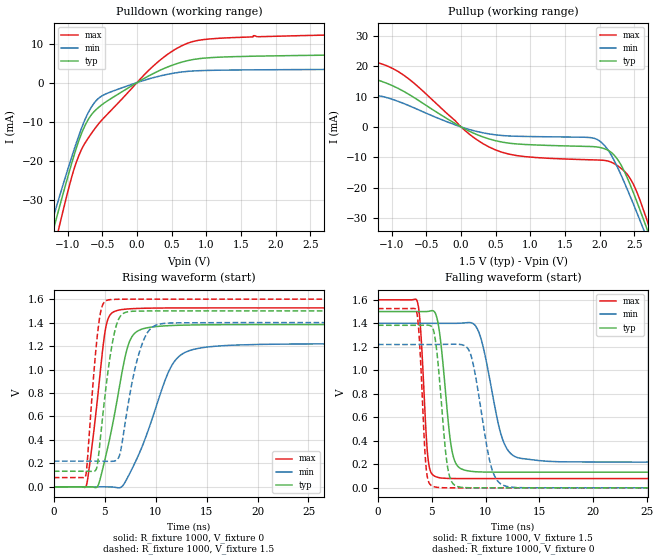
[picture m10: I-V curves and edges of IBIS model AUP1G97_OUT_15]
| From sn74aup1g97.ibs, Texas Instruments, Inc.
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[Model]   AUP1G97_OUT_15
Model_type  Output
Vref =   0
Rref =   1E6
Cref =   30p
Vmeas =   0.75
| variable   typ   min   max
C_comp   2.79pF   1.99pF   4.00pF
| C_pullup   3.03pF   1.99pF   4.00pF
| C_pulldown   2.56pF   2.15pF   3.05pF
[Temperature Range]   40   100   -40
| Ambient temperature   25   85   -40
[Voltage range]   1.5   1.4   1.6
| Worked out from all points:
|   slope of the pulldown table from 0 to 0.225 V, typ, clamps not added: 101 ohm
|   slope of the pullup table from 0 to 0.225 V, typ, clamps not added: 90.4 ohm
|   rising waveform, R_fixture 1000, V_fixture 0: 20-80 % time 1.86ns typ, 3.07ns min, 1.18ns max; typ from 0 V to 1.38 V
|   falling waveform, R_fixture 1000, V_fixture 1.5: 20-80 % time 873ps typ, 1.57ns min, 528ps max; typ from 1.5 V to 0.133 V
|   rising waveform, R_fixture 1000, V_fixture 1.5: 20-80 % time 1.19ns typ, 1.61ns min, 854ps max; typ from 0.133 V to 1.5 V
|   falling waveform, R_fixture 1000, V_fixture 0: 20-80 % time 790ps typ, 1.33ns min, 489ps max; typ from 1.38 V to 0 V
[Pulldown]
| AUP1G97_OUT_15
|   Voltage   I(typ)   I(min)   I(max)
-3.6V     -206.1mA   -188.4mA   -227.8mA
-1.265V   -41.59mA   -37.94mA   -47.65mA
-1.21V    -37.9mA    -34.62mA   -43.48mA
-1.11V    -31.29mA   -28.67mA   -36mA
-945mV    -20.84mA   -19.21mA   -24.37mA
-855mV    -15.7mA    -14.39mA   -19.43mA
-720mV    -9.972mA   -8.297mA   -14.65mA
-570mV    -6.595mA   -4.269mA   -10.91mA
260mV     2.544mA    1.373mA    4.642mA
810mV     5.906mA    2.979mA    10.53mA
1.685V    6.762mA    3.268mA    12.01mA
7.2V      7.827mA    3.609mA    13.77mA
[Pullup]
| AUP1G97_OUT_15
|   Voltage   I(typ)   I(min)   I(max)
-3.6V     29.66mA    17.95mA    40.7mA
-2.925V   22.54mA    13.64mA    31.9mA
-2.13V    15.77mA    9.503mA    23.16mA
-1.025V   13.91mA    9.322mA    19.64mA
130mV     -1.525mA   -910.1uA   -2.565mA
590mV     -4.979mA   -2.819mA   -8.32mA
1.925V    -6.506mA   -3.765mA   -10.85mA
2.175V    -8.513mA   -9.57mA    -11.67mA
2.395V    -16.55mA   -20.31mA   -15.49mA
2.615V    -29.32mA   -32.63mA   -26.15mA
2.72V     -35.89mA   -38.74mA   -33.2mA
7.2V      -352.6mA   -330.3mA   -379.5mA
[Ramp]
| AUP1G97_OUT_15
| variable   typ   min   max
dV/dt_r   0.83/1.87E-09   0.74/3.09E-09   0.92/1.18E-09
dV/dt_f   0.83/8.80E-10   0.71/1.58E-09   0.92/5.34E-10
R_load = 1000
[Rising Waveform]
| AUP1G97_OUT_15
R_fixture =   1000
C_fixture =   0
L_fixture =   0
V_fixture =   0
V_fixture_min = 0
V_fixture_max = 0
|   Time   V(typ)   V(min)   V(max)
0s        16.57nV    92.2nV     986.7pV
3.18ns    358.5uV    -8.611uV   7.778mV
4.285ns   3.073mV    321.5uV    749.9mV
5.015ns   232.1mV    393.9uV    1.316V
5.895ns   588.2mV    -2.299mV   1.493V
7.04ns    1.124V     47.07mV    1.514V
7.78ns    1.293V     172.1mV    1.519V
11.27ns   1.374V     981.9mV    1.525V
12.91ns   1.379V     1.147V     1.525V
34.99ns   1.383V     1.22V      1.525V
[Falling Waveform]
| AUP1G97_OUT_15
R_fixture =   1000
C_fixture =   0
L_fixture =   0
V_fixture =   1.5
V_fixture_min = 1.4
V_fixture_max = 1.6
|   Time   V(typ)   V(min)   V(max)
0s        1.5V       1.4V       1.6V
3.655ns   1.5V       1.4V       1.588V
4.635ns   1.501V     1.4V       269.1mV
5.31ns    1.49V      1.4V       97.66mV
6.825ns   346.1mV    1.4V       79.77mV
7.735ns   161.9mV    1.401V     79.22mV
9.36ns    136mV      1.329V     79.09mV
11.43ns   133.4mV    456.2mV    79.08mV
12.77ns   133.2mV    264.6mV    79.08mV
34.99ns   133.1mV    219.3mV    79.08mV
[Rising Waveform]
| AUP1G97_OUT_15
R_fixture =   1000
C_fixture =   0
L_fixture =   0
V_fixture =   1.5
V_fixture_min = 1.4
V_fixture_max = 1.6
|   Time   V(typ)   V(min)   V(max)
0s        133.1mV    219.3mV    79.08mV
3.125ns   133.3mV    219.4mV    93.83mV
4.23ns    169.6mV    219.4mV    1.256V
4.635ns   468mV      219mV      1.506V
5.135ns   859.8mV    217.9mV    1.587V
5.845ns   1.271V     218.7mV    1.598V
6.49ns    1.449V     280.1mV    1.599V
8.245ns   1.498V     1.102V     1.6V
9.965ns   1.499V     1.376V     1.6V
34.99ns   1.5V       1.4V       1.6V
[Falling Waveform]
| AUP1G97_OUT_15
R_fixture =   1000
C_fixture =   0
L_fixture =   0
V_fixture =   0
V_fixture_min = 0
V_fixture_max = 0
|   Time   V(typ)   V(min)   V(max)
0s        1.383V     1.22V      1.525V
3.565ns   1.383V     1.22V      1.51V
4.465ns   1.385V     1.22V      188.4mV
5.03ns    1.369V     1.22V      16.01mV
6.44ns    197.4mV    1.221V     340.7uV
7.235ns   16.9mV     1.222V     47.73uV
8.615ns   768uV      1.137V     3.702uV
10.43ns   43.86uV    214mV      287.6nV
11.61ns   10.37uV    23.19mV    172.9nV
34.99ns   -39.23nV   51.17nV    -88.64nV
